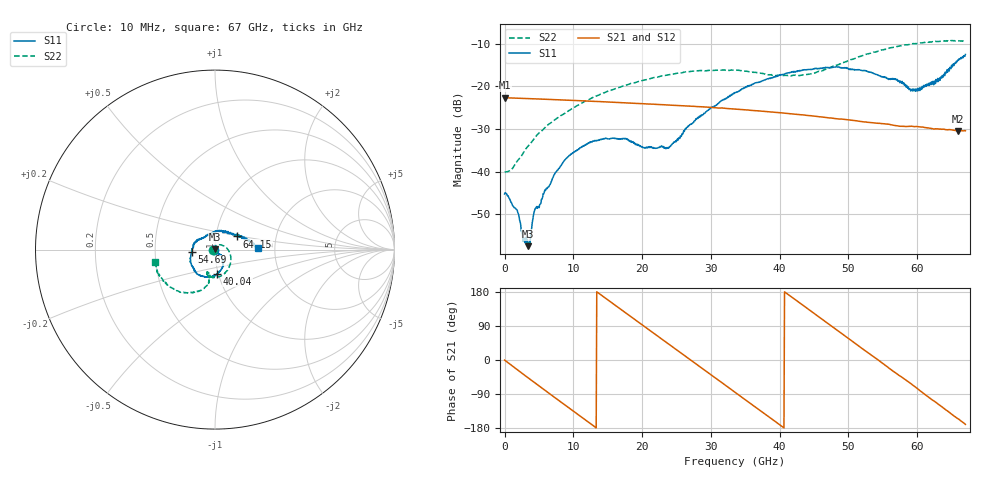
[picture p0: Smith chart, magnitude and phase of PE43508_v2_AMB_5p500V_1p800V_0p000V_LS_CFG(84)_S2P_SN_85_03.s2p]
!Keysight Technologies,N5227A,US51270237,A.10.43.00
!Date: Wednesday, August 22, 2018 17:15:25
!Correction: S11(Full 2 Port(1,3))
!S31(Full 2 Port(1,3))
!S13(Full 2 Port(1,3))
!S33(Full 2 Port(1,3))
!S2P File: Measurements: S11, S31, S13, S33:
# Hz S  dB  R 50
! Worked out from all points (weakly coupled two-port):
!   801 points, 10 MHz to 67 GHz, reference 50 ohm
!   highest |S21| = -22.64 dB at 10 MHz (marker M1); lowest = -30.4 dB at 65.91 GHz (marker M2)
!   lowest |S11| = -57.5 dB at 3.443 GHz (marker M3), VSWR 1.00, Z = 50.1 + j0.112 ohm
!   |S11| at or under -10 dB: start of sweep to end of sweep
!   |S22| runs from -40.1 to -9.2 dB; largest |S21 - S12| = 0.00037
!   S11 on the Smith chart (normalised r, x): 10 MHz: 0.99, -0.00; 40.04 GHz: 0.99, -0.27; 54.69 GHz: 0.77, -0.02; 64.15 GHz: 1.26, +0.19; 67 GHz: 1.62, +0.03
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1e7  -45.23 -176.6  -22.64 -0.3  -22.64 -0.2  -40.12 -179.4
1.768488e9  -48.91 150.6  -22.77 -24.5  -22.77 -24.5  -37.69 116.7
2.6896e9  -56.23 119.0  -22.82 -37.1  -22.82 -37.1  -35.73 95.2
3.443238e9  -57.49 56.7  -22.87 -47.3  -22.88 -47.3  -34.00 82.6
4.36435e9  -49.17 5.2  -22.92 -59.6  -22.93 -59.6  -32.15 69.6
5.955362e9  -44.43 -21.5  -23.02 -81.0  -23.02 -81.0  -29.56 53.7
8.802438e9  -37.21 -55.1  -23.21 -119.0  -23.21 -119.0  -26.30 28.6
1.123082e10  -34.12 -68.8  -23.38 -151.3  -23.39 -151.3  -23.93 9.1
1.583639e10  -32.18 -91.6  -23.73 147.7  -23.73 147.8  -20.68 -20.8
2.236791e10  -34.32 -78.2  -24.25 61.6  -24.25 61.6  -17.75 -55.3
2.395892e10  -34.28 -60.9  -24.39 40.7  -24.39 40.7  -17.24 -62.4
2.81458e10  -27.49 -43.1  -24.75 -14.5  -24.75 -14.4  -16.32 -80.3
3.3505e10  -21.52 -58.2  -25.32 -85.3  -25.33 -85.4  -16.21 -100.1
4.003652e10  -17.41 -84.7  -26.18 -171.4  -26.17 -171.3  -17.39 -109.2
4.472582e10  -15.98 -107.5  -26.90 126.6  -26.89 126.6  -17.01 -102.2
4.841028e10  -15.43 -126.6  -27.61 77.9  -27.61 77.9  -14.98 -100.4
5.469059e10  -17.69 -173.2  -28.71 -5.2  -28.68 -5.4  -11.54 -116.0
5.586291e10  -18.39 173.2  -28.87 -21.2  -28.87 -21.6  -11.04 -120.5
6.004979e10  -20.49 108.2  -29.43 -75.9  -29.44 -76.3  -9.93 -137.4
6.415292e10  -16.91 30.7  -30.16 -131.6  -30.22 -131.8  -9.34 -154.9
6.591141e10  -13.81 12.6  -30.44 -154.8  -30.53 -154.9  -9.28 -162.2
6.7e10  -12.51 2.1  -30.41 -170.0  -30.48 -170.0  -9.31 -168.1
